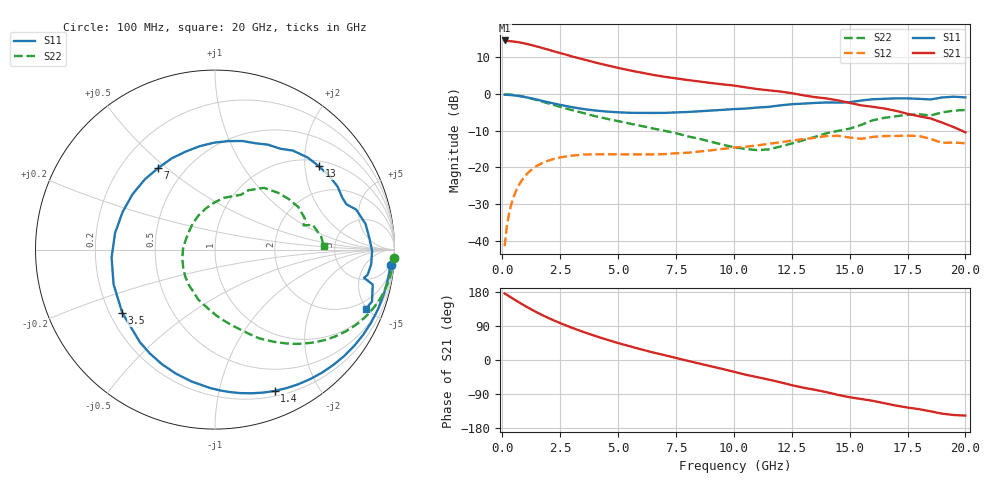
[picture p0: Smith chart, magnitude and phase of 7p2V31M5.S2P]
! Infineon Technologies  Discrete & RF Semiconductors
! bfp620
! VCE =  2.3 V,  IC =  1.5 mA
! Common Emitter S-Parameters:  Sep 2002
# GHz  S  MA  R  50
!  f  S11  S21  S12  S22
! GHz  MAG  ANG  MAG  ANG  MAG  ANG  MAG  ANG
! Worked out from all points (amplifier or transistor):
!   59 points, 100 MHz to 20 GHz, reference 50 ohm
!   highest |S21| = 14.6 dB at 100 MHz (marker M1)
!   |S21| within 3 dB of that: start of sweep to 2.25 GHz
!   unconditionally stable (mu >= 1): 5.995 GHz to 15.66 GHz; 17.79 GHz to 19.14 GHz; 19.53 GHz to end of sweep
!   at 1 GHz: K = 0.13, MSG = 18.0 dB, |S12| = -22.3 dB
!   at 5.5 GHz: K = 0.92, MSG = 11.5 dB, |S12| = -16.5 dB
!   at 20 GHz: K = 1.29, MAG = -1.7 dB, |S12| = -13.4 dB
!   S11 on the Smith chart (normalised r, x): 100 MHz: 4, -22; 1.4 GHz: 0.25, -1.48; 3.5 GHz: 0.25, -0.29; 7 GHz: 0.36, +0.47; 13 GHz: 1.15, +2.36; 20 GHz: 1.37, -4.87
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0.1  0.9824 -5.0  5.399 175.7  0.0084 84.3  0.9967 -2.7
0.2  0.9771 -10.1  5.339 171.9  0.0161 82.5  0.9937 -5.4
0.4  0.967 -20.1  5.255 164.2  0.0323 78.0  0.9816 -10.8
0.8  0.9324 -39.5  5.04 149.2  0.0634 66.5  0.9379 -20.8
1.1  0.8956 -53.6  4.805 138.7  0.0834 57.7  0.8931 -27.7
1.4  0.8547 -67.1  4.546 128.7  0.1001 49.6  0.8434 -33.8
1.9  0.7849 -88.0  4.114 113.5  0.1207 38.0  0.7607 -42.7
2.4  0.7243 -107.6  3.705 99.9  0.1344 28.4  0.6848 -50.1
3  0.664 -129.1  3.276 85.2  0.1444 18.6  0.6057 -57.8
3.5  0.6254 -145.7  2.978 74.1  0.1495 11.9  0.5519 -63.6
4  0.5972 -161.1  2.709 63.7  0.1508 5.9  0.5006 -68.6
5  0.5644 170.6  2.282 44.8  0.1509 -2.2  0.4282 -78.0
6  0.5535 146.1  1.967 28.0  0.1501 -7.7  0.3679 -88.7
7  0.5539 124.8  1.725 12.9  0.1516 -10.9  0.3161 -100.6
8.5  0.5824 98.4  1.488 -9.2  0.1643 -15.1  0.2459 -125.9
10.5  0.6343 69.0  1.238 -38.7  0.1915 -25.1  0.1785 179.0
12  0.7019 51.8  1.085 -58.7  0.2192 -32.8  0.192 129.9
13  0.742 38.7  0.963 -73.1  0.2427 -41.0  0.2348 102.6
13.5  0.7574 32.9  0.909 -78.6  0.2536 -45.7  0.2604 91.5
15  0.7748 19.0  0.759 -98.3  0.2555 -65.2  0.3375 64.7
17  0.8756 -0.5  0.591 -120.3  0.2682 -79.3  0.4989 34.2
20  0.9019 -21.6  0.301 -146.7  0.2133 -104.7  0.6068 1.7
